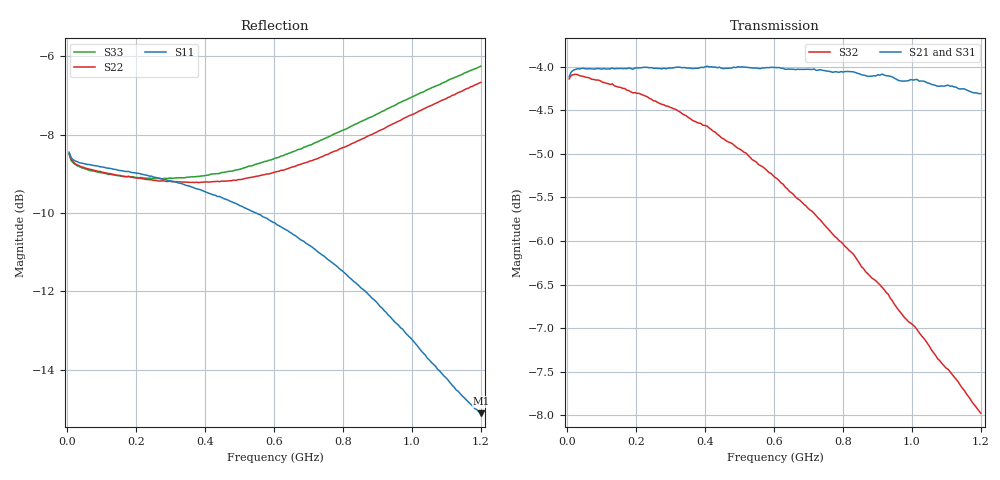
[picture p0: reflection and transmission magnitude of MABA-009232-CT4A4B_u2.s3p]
#	MHz	S	dB	R	50
!FREQ	R1	I1	R2	I2	R3	I3
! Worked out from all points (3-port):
!   201 points, 5 MHz to 1.2 GHz, reference 50 ohm
!   strongest paths, dB at 5 MHz, 303.8 MHz, 602.5 MHz, 901.2 MHz, 1.2 GHz:
!     S21: -4.1, -4.0, -4.0, -4.1, -4.3
!     S31: -4.1, -4.0, -4.1, -4.2, -4.5
!     S32: -4.1, -4.5, -5.3, -6.5, -8.0
!   lowest |S11| = -15.1 dB at 1.2 GHz (marker M1), VSWR 1.43, Z = 53.6 + j18.1 ohm
!   |S11| at or under -10 dB: 547.4 MHz to end of sweep
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5  -8.45 175.4  -4.11 -177.9  -4.10 2.1
   -4.11 -177.9  -8.48 174.5  -4.14 -178.5
   -4.10 2.1  -4.14 -178.5  -8.49 174.5
52.8  -8.75 175.9  -4.02 176.2  -4.02 -3.3
      -4.02 176.1  -8.86 168.1  -4.12 172.0
      -4.02 -3.3  -4.12 171.9  -8.87 167.6
160.35  -8.92 170.0  -4.03 167.4  -4.00 -11.2
        -4.02 167.5  -9.06 147.5  -4.25 155.5
        -4.00 -11.2  -4.25 155.6  -9.07 146.1
321.675  -9.23 160.5  -4.02 154.6  -4.01 -22.8
         -4.00 154.5  -9.21 116.3  -4.52 131.5
         -4.01 -22.8  -4.51 131.4  -9.10 114.0
447.15  -9.60 152.5  -4.01 144.6  -4.01 -31.9
        -4.02 144.5  -9.19 92.5  -4.80 113.2
        -4.01 -31.9  -4.82 113.1  -8.97 89.8
602.5  -10.26 141.4  -4.01 132.4  -4.05 -43.3
       -4.01 132.1  -8.95 63.7  -5.25 91.3
       -4.05 -43.3  -5.27 91.1  -8.60 61.2
763.825  -11.24 127.7  -4.04 119.6  -4.13 -55.3
         -4.05 119.4  -8.46 36.2  -5.85 69.2
         -4.13 -55.3  -5.89 69.0  -8.03 34.5
919.175  -12.49 111.4  -4.09 107.5  -4.24 -66.8
         -4.09 107.2  -7.85 12.9  -6.52 49.0
         -4.24 -66.8  -6.56 48.8  -7.39 11.8
1038.675  -13.63 95.9  -4.13 98.2  -4.34 -75.9
          -4.17 98.0  -7.32 -2.7  -7.07 34.0
          -4.34 -75.9  -7.14 34.0  -6.88 -3.3
1200  -15.12 68.8  -4.24 85.8  -4.52 -88.1
      -4.31 85.9  -6.66 -21.0  -7.88 14.9
      -4.52 -88.1  -7.98 15.3  -6.25 -21.0
